(* Logix 5000 DataType export UDT_C30S_DN; software revision 20.01 *)

TYPE UDT_PLC_To_C30S :   // Output from PLC
STRUCT
   Automatic : BOOL;
   Start : BOOL;
   AckFault : BOOL;
   DS1 : BOOL;
   DS2 : BOOL;
   ExtDigSig : BOOL;
   Res1 : BOOL;
   Res2 : BOOL;
   Prog : SINT;
END_STRUCT
END_TYPE

TYPE UDT_C30S_To_PLC :   // Input to PLC
STRUCT
   NoFault : BOOL;
   ReadyToStart : BOOL;
   OK : BOOL;
   NOK : BOOL;
   DepthReached : BOOL;
   Res1 : BOOL;
   Res2 : BOOL;
   Res3 : BOOL;
   ProgResult : SINT;
   StrategyResult : SINT;
   CodeResult : INT;
   TorqueResult : REAL;
   PreTorqueResult : REAL;
   AngleResult : REAL;
   DepthResult : REAL;
   DriveTime : REAL;
   CycleNumber : DINT;
END_STRUCT
END_TYPE

TYPE UDT_C30S_DN :   // In and Output Data for Weber C30S
STRUCT
   OUT : UDT_PLC_To_C30S;   // Output Data
   IN : UDT_C30S_To_PLC;   // Input Data
   Temp_In : SINT[29];
   Temp_Out : SINT[2];
END_STRUCT
END_TYPE
